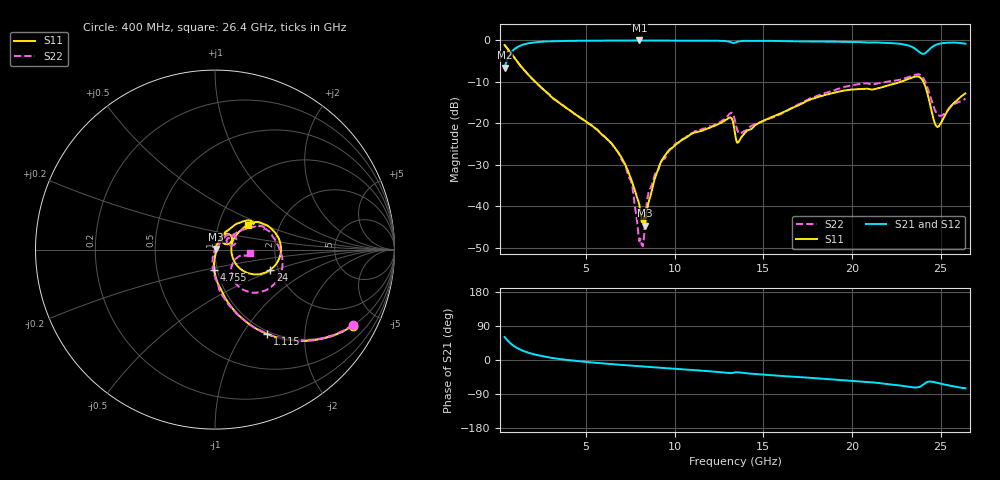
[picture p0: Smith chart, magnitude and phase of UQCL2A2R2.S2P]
! AVX Corporation
! Date:  10/27/06
! Part No:  UQCL2A2R2
! Description:  Ultra Low ESR Microwave capacitors
! Mounting Orientation:  Horizontal
# GHZ S DB R 50
! Freq  |S11|  S11 Ph  |S21|  S21 Ph  |S12|  S12 Ph  |S22|  S22 Ph
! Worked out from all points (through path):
!   401 points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, 400 MHz to 26.4 GHz, reference 50 ohm
!   highest |S21| = -0.02 dB at 8.005 GHz (marker M1); lowest = -6.6 dB at 400 MHz (marker M2)
!   group delay of S21, straight-line fit = 10.1 ps
!   lowest |S11| = -44.6 dB at 8.33 GHz (marker M3), VSWR 1.01, Z = 50.4 + j0.411 ohm
!   |S11| at or under -10 dB: 2.136 GHz to 22.73 GHz (20.59 GHz wide, 166 % of centre); 24.03 GHz to end of sweep
!   |S22| runs from -49.6 to -1.1 dB; largest |S21 - S12| = 0.0032
!   S11 on the Smith chart (normalised r, x): 400 MHz: 0.99, -3.64; 1.115 GHz: 0.96, -1.30; 4.755 GHz: 0.97, -0.22; 24 GHz: 1.81, -0.46; 26.4 GHz: 1.38, +0.40
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0.4  -1.13 -28.8  -6.58 60.6  -6.58 60.6  -1.14 -28.6
1.115  -5.14 -58.3  -1.63 31.5  -1.64 31.4  -5.14 -58.0
2.285  -10.62 -76.8  -0.40 12.6  -0.41 12.6  -10.62 -77.6
4.755  -18.82 -91.5  -0.09 -4.0  -0.09 -3.9  -18.89 -95.2
7.095  -28.99 -89.4  -0.05 -13.3  -0.04 -13.3  -29.31 -109.8
7.55  -33.56 -80.0  -0.04 -14.9  -0.04 -14.9  -34.09 -111.5
8.005  -39.62 -50.6  -0.02 -16.6  -0.02 -16.6  -48.40 -55.2
8.135  -43.68 -26.9  -0.04 -17.1  -0.03 -17.1  -49.23 7.8
8.33  -44.59 43.8  -0.05 -17.8  -0.04 -17.7  -42.62 8.2
8.59  -38.00 56.8  -0.06 -18.6  -0.06 -18.6  -35.84 43.1
9.11  -30.49 69.7  -0.06 -20.4  -0.05 -20.3  -30.67 49.8
9.695  -26.35 64.3  -0.06 -22.1  -0.05 -22.1  -26.43 56.0
10.995  -22.39 62.1  -0.07 -26.4  -0.06 -26.4  -22.31 54.4
13.075  -18.64 45.9  -0.31 -34.5  -0.30 -34.5  -17.77 40.2
13.4  -22.41 22.9  -0.57 -32.6  -0.56 -32.6  -19.33 13.6
13.79  -23.14 59.0  -0.16 -33.7  -0.15 -33.7  -22.20 33.2
17.755  -14.07 48.2  -0.26 -47.4  -0.25 -47.5  -13.77 34.0
22.11  -10.75 31.6  -0.64 -63.7  -0.63 -63.8  -9.87 17.4
23.28  -9.15 15.3  -1.38 -71.2  -1.37 -71.3  -8.72 -2.3
23.995  -9.68 -20.2  -3.25 -65.6  -3.24 -65.8  -8.85 -39.3
24.84  -20.85 1.8  -0.91 -60.7  -0.89 -60.8  -17.90 -41.6
26.4  -12.76 37.0  -0.81 -74.6  -0.80 -74.8  -14.03 -6.3
